(*此PLC项目为FB_XmlSrvWrite对应例程,FB_XmlSrvRead请打开名称为XML Read的PLC项目*)
PROGRAM MAIN
VAR
	ST_XmlWrite1: ST_XmlTest1;
	FB_XmlWrite: FB_XmlSrvWrite;
	b_Execute: BOOL;
	sFilePath: T_MaxString:='Hard Disk\temp\Test.xml';		//XML文件生成的路径
	sXPath: T_MaxString:='/dataentry/MAIN.ST_XmlWrite1';	//要从XML文档中写入数据的标记地址,一般为固定/dataentry开头+主逻辑中需要写入的变量，即MAIN.变量名
END_VAR

FB_XmlWrite(
	sNetId:= , 							//默认为本地的NetId,连接控制器后使用的是控制器本地的编程环境，也可以不填写
	ePath:= PATH_GENERIC, 				//用于在目标设备上选择用于打开文件的TwinCAT系统路径,PATH_GENERIC即表示在选定/通用文件夹中搜索/打开/创建文件
	nMode:= XMLSRV_ADDMISSING, 			//用于控制XML文件的计算方式,具体解释可参考文档说明
	pSymAddr:= ADR(ST_XmlWrite1), 		//将XML文件中的数据写入的PLC变量的地址
	cbSymSize:= SIZEOF(ST_XmlWrite1), 	//将XML文件中的数据写入的PLC变量的大小
	sFilePath:= sFilePath, 				
	sXPath:= sXPath, 
	bExecute:= b_Execute, 				//功能块触发条件，置TRUE则执行一次
	tTimeout:= , 						//功能块执行的最大时间，超时报错
	bBusy=> , 
	bError=> , 
	nErrId=> );

END_PROGRAM
